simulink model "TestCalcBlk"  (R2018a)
settings: Solver=ode15s  StartTime=0.0  StopTime=150  MaxStep=0.1  RelTol=1e-5
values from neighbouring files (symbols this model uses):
  d0 = [Fh, Tcin, Thin]    [Main.m]    (also in Main_OL.m; runTestCalcBlk.m; runTransf.m = [Fh; Tcin; U0; Ffeed0; m0; Tfeed0]; runTransfOL.m)
  d_step = [Fh, Tcin+0, Thin*1]    [Main_OL.m]    (also in runTestCalcBlk.m = [Fh, Tcin, Thin]; Main.m = [Fh, Tcin, Thin])
  d_tstep = 300    [Main.m]    (also in Main_OL.m = 3000; runTestCalcBlk.m; runTransf.m = [500; 50000; 70000; 130000; 50000; 50000]; runTransfOL.m = [500 5000 7000 13000])
  Fc0 = 5    [Main.m]    (also in Main_OL.m; runTestCalcBlk.m; runTransf.m; runTransfOL.m)
  nd = size(d0,2)    [Main.m]    (also in Main_OL.m; runTestCalcBlk.m; runTransf.m = size(d0,1); runTransfOL.m)
  np = size(p,2)    [Main.m]    (also in Main_OL.m; runTestCalcBlk.m; runH2Psim.m = length(param); runTransf.m)
  nu = 1    [Main.m]    (also in Main_OL.m; runTestCalcBlk.m; runH2Psim.m = length(u0); runTransf.m)
  p = [N, Fc0, rhoc, rhoh,U,A,cpc,cph]    [Main.m]    (also in Main_OL.m; runTestCalcBlk.m; NonlinearMap.m = [U;A;Fc(i);Fh;cpc;cph;Tcin;Thin]; runTransf.m = [N, Fc0, rhoc, rhoh, U0, A,cpc,cph])
  Thsp = Thsp0+dThsp    [Main.m]    (also in Main_OL.m = sp(j); runTestCalcBlk.m; runTransf.m = Thsp0; runTransfOL.m = Thsp0)
  Thsp0 = Thend(end)    [Main.m]    (also in Main_OL.m; runTestCalcBlk.m; runTransf.m = x0(end-1);  2.971202611676064e+02; runTransfOL.m = x0(end);  2.971202611676064e+02)
undefined symbols (not defined in the file or in its folder): calcblock, calcblock2

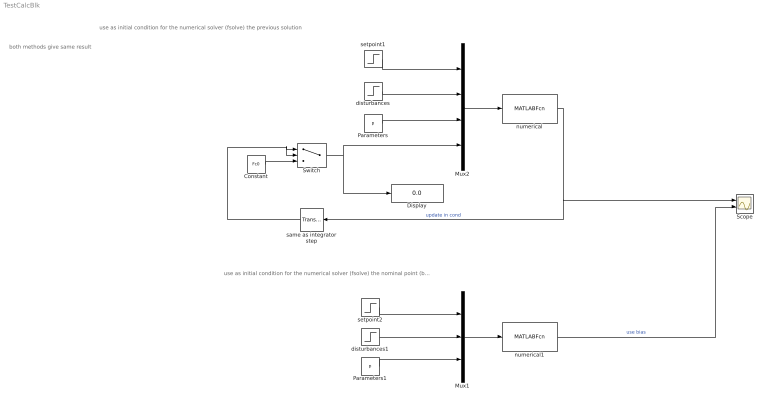
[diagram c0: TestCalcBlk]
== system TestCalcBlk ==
  note: use as initial condition for the numerical solver (fsolve) the nominal point (bias)
  note: use as initial condition for the numerical solver (fsolve) the previous solution
  note: both methods give same result
  Constant : Constant  Value=Fc0
  Display : Display
  Mux1 : Mux  Inputs=3
  Mux2 : Mux
  Parameters : Constant  Value=p
  Parameters1 : Constant  Value=p
  Scope : Scope  NumInputPorts=2
  Switch : Switch  Criteria=u2 > Threshold  Threshold=3
  disturbances : Step  Time=d_tstep  Before=d0  After=d_step  SampleTime=0
  disturbances1 : Step  Time=d_tstep  Before=d0  After=d_step  SampleTime=0
  numerical : MATLABFcn  MATLABFcn=calcblock2(u(nu),u(nu+1:nu+nd),u(nu+nd+1:nu+nd+np),u(nu+nd+np+1))
  numerical1 : MATLABFcn  MATLABFcn=calcblock(u(nu),u(nu+1:nu+nd),u(nu+nd+1:nu+nd+np))
  same as integrator step : TransportDelay  DelayTime=0.2
  setpoint1 : Step  Time=10  Before=Thsp0  After=Thsp  SampleTime=0
  setpoint2 : Step  Time=10  Before=Thsp0  After=Thsp  SampleTime=0
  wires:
  Parameters/1 -> Mux2/3
  disturbances/1 -> Mux2/2
  Mux2/1 -> numerical/1
  setpoint1/1 -> Mux2/1
  numerical/1 -> same as integrator step/1, Scope/1  "update in cond"
  setpoint2/1 -> Mux1/1
  Parameters1/1 -> Mux1/3
  Mux1/1 -> numerical1/1
  disturbances1/1 -> Mux1/2
  Constant/1 -> Switch/3
  Switch/1 -> Mux2/4, Display/1
  same as integrator step/1 -> Switch/2, Switch/1
  numerical1/1 -> Scope/2  "use bias"
